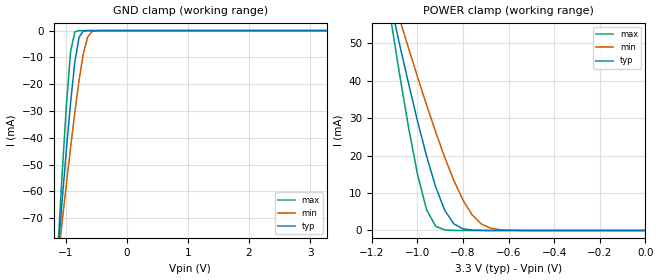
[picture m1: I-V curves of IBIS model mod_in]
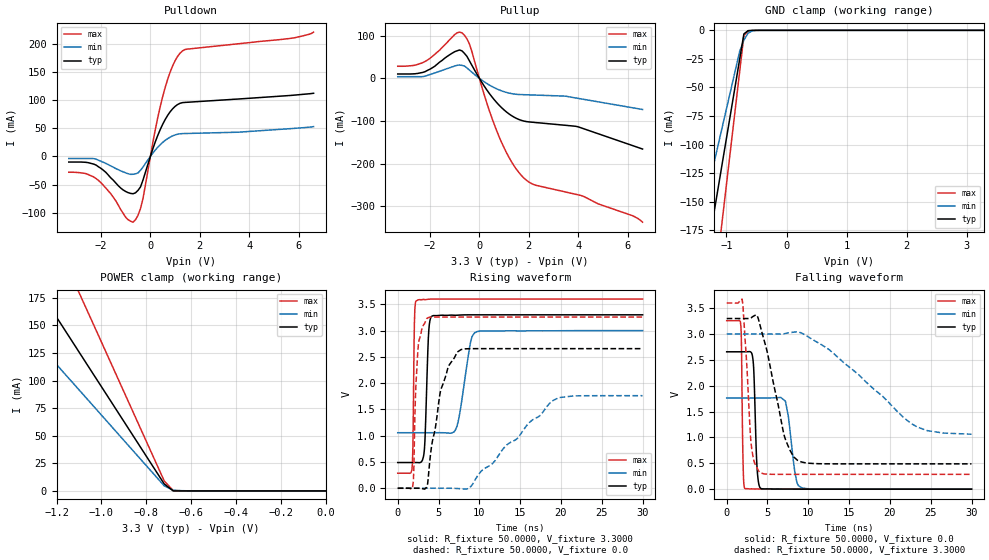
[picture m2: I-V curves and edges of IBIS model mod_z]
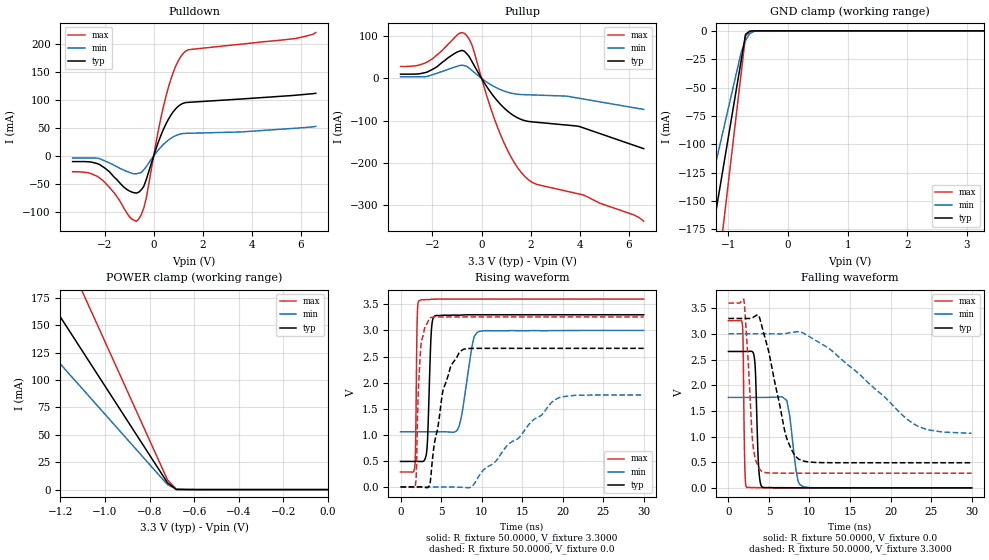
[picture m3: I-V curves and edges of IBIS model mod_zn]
| IBIS (I/O, Buffer, Information, Specification) Model, officially
| electronic behavioral standard for Buffer structures of digital pins.
[IBIS ver]  4.0
[File name] 54ac151_3v3_rev1.ibs
[File Rev]  1.0
[Date]   9 Oct 2020
[Source]   CAD & Design Services (Catania) - STMicroelectronics
[Notes]
  (Note1) This IBIS model is the model of the product with package
   (Flat16 package elements);
  (Note2) This IBIS model is extracted with nominal 3.3V power supply
   (min:3.0V, typ:3.3V, max:3.6V);
  (Note3) This model has few Warnings about the non-monotonicity
   of I-V curves, but they are not indicative of problems
   inside the model;
[Copyright] (c) 2020 STMicroelectronics
|   Component 54AC151
[Component] 54AC151
[Manufacturer] STMicroelectronics
[Package]
| variable  typ   min   max
R_pkg   0.0   0.0   0.0
L_pkg   0.0H   0.0H   0.0H
C_pkg   0.0F   0.0F   0.0F
[Pin]   signal_name   model_name   R_pin   L_pin   C_pin
1   I3   mod_in   87.8m   2.68nH   1.16pF
2   I2   mod_in   53.6m   1.94nH   1.11pF
3   I1   mod_in   34.1m   1.02nH   0.87pF
4   IO   mod_in   34.1m   1.02nH   0.87pF
5   Z   mod_z   34.1m   1.02nH   0.87pF
6   ZN   mod_zn   34.1m   1.02nH   0.87pF
7   EN   mod_en   53.6m   1.94nH   1.11pF
8   GND   GND   87.8m   2.68nH   1.16pF
9   S2   mod_s   87.8m   2.68nH   1.16pF
10   S1   mod_s   53.6m   1.94nH   1.11pF
11   S0   mod_s   34.1m   1.02nH   0.87pF
12   I7   mod_in   34.1m   1.02nH   0.87pF
13   I6   mod_in   34.1m   1.02nH   0.87pF
14   I5   mod_in   34.1m   1.02nH   0.87pF
15   I4   mod_in   53.6m   1.94nH   1.11pF
16   VCC   POWER   87.8m   2.68nH   1.16pF
| Models and submodels in the file (5): mod_in (Input), mod_z (3-state), mod_zn (3-state), mod_en (Input), mod_s (Input)
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|   Model mod_in
[Model]   mod_in
Model_type Input
Vinl   =   0.8000V
Vinh   =   2.0000V
C_comp   0.584pF   0.423pF   0.735pF
[Temperature Range]  25.0000   0.1250k   -55.0000
[Voltage Range]   3.3000V   3.0000V   3.6000V
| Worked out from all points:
|   GND clamp passes 1 mA (typ) near -0.74 V on its own axis
|   POWER clamp passes 1 mA (typ) near -0.82 V on its own axis
[GND_clamp]
|Voltage   I(typ)   I(min)   I(max)
-3.3V     -749mA     -568.4mA   -1.036A
-1.13V    -83.59mA   -86.24mA   -82mA
-1.06V    -63.75mA   -71.67mA   -54.05mA
-990mV    -44.61mA   -57.39mA   -28.12mA
-920mV    -26.72mA   -43.53mA   -7.665mA
-850mV    -11.52mA   -30.34mA   -438.9uA
-780mV    -2.357mA   -18.3mA    -11.16uA
-710mV    -202.6uA   -8.403mA   -269.9nA
-640mV    -13.61uA   -2.366mA   -6.525nA
-570mV    -893.7nA   -396.6uA   -166.8pA
-430mV    -3.851nA   -7.049uA   -9.012pA
3.28V     6.52pA     5.985nA    5.92pA
[POWER_clamp]
|Voltage   I(typ)   I(min)   I(max)
-3.28V    721.1mA    542.9mA    1.005A
-1.12V    61.08mA    64.91mA    57.6mA
-1.08V    50.1mA     56.8mA     42.24mA
-1.04V    39.44mA    48.83mA    27.8mA
-1V       29.27mA    41.04mA    15.03mA
-960mV    19.83mA    33.48mA    5.53mA
-920mV    11.6mA     26.24mA    1.117mA
-880mV    5.323mA    19.44mA    149.5uA
-840mV    1.752mA    13.28mA    18.09uA
-760mV    95.85uA    4.147mA    257.2nA
-680mV    4.309uA    632.9uA    3.657nA
0V        6.6pA      45.39pA    7.2pA
|   Model mod_z
[Model]   mod_z
Model_type 3-state
Polarity   Non-Inverting
Enable   Active-Low
| Vinl   =   0.8000V
| Vinh   =   2.0000V
Vmeas  =   1.650V
Cref   =   50pF
Rref   =   500
Vref   =   0.0
C_comp   3.207pF   2.433pF   4.228pF
[Temperature Range]  25.0000   0.1250k   -55.0000
[Voltage Range]   3.3000V   3.0000V   3.6000V
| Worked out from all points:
|   slope of the pulldown table from 0 to 0.495 V, typ, clamps not added: 8.73 ohm
|   slope of the pullup table from 0 to 0.495 V, typ, clamps not added: 11.6 ohm
|   GND clamp passes 1 mA (typ) near -0.66 V on its own axis
|   POWER clamp passes 1 mA (typ) near -0.69 V on its own axis
|   rising waveform, R_fixture 50.0000, V_fixture 3.3000: 20-80 % time 350ps typ, 1.11ns min, 147ps max; typ from 0.489 V to 3.3 V
|   rising waveform, R_fixture 50.0000, V_fixture 0.0: 20-80 % time 1.92ns typ, 7.15ns min, 456ps max; typ from 0 V to 2.66 V
|   falling waveform, R_fixture 50.0000, V_fixture 0.0: 20-80 % time 316ps typ, 778ps min, 163ps max; typ from 2.66 V to 0 V
|   falling waveform, R_fixture 50.0000, V_fixture 3.3000: 20-80 % time 2.19ns typ, 8.06ns min, 717ps max; typ from 3.3 V to 0.489 V
[Pulldown]
|Voltage   I(typ)   I(min)   I(max)
-3.3V     -10.02mA   -3.72mA    -28.12mA
-2.1V     -18.41mA   -6.713mA   -42.56mA
-1.6V     -38.11mA   -16.98mA   -66.25mA
-1V       -62.22mA   -29.14mA   -107.8mA
-700mV    -66.24mA   -31.66mA   -116.7mA
-500mV    -60.23mA   -29.28mA   -104.6mA
-300mV    -42.06mA   -19.04mA   -75.1mA
200mV     25.93mA    11.34mA    47.73mA
600mV     65.52mA    28.45mA    122.5mA
900mV     84.46mA    36.38mA    160.6mA
1.2V      94.2mA     40.13mA    183.1mA
6.6V      112mA      52.87mA    220.5mA
[Pullup]
|Voltage   I(typ)   I(min)   I(max)
-3.3V     10.02mA    3.72mA     28.12mA
-2.2V     15.31mA    4.805mA    39.21mA
-1V       62.21mA    28.63mA    102.3mA
-700mV    64.18mA    30.12mA    106.5mA
-400mV    40.78mA    19.13mA    80.3mA
300mV     -27.16mA   -12.16mA   -57.61mA
800mV     -63.16mA   -27.27mA   -137.1mA
1.3V      -87.59mA   -35.96mA   -195.8mA
1.7V      -98.8mA    -38.31mA   -227.9mA
2.2V      -103.4mA   -39.31mA   -249.4mA
4V        -114mA     -47.24mA   -273.5mA
6.6V      -166mA     -73.24mA   -337.6mA
[GND_clamp]
|Voltage   I(typ)   I(min)   I(max)
-3.3V     -818.6mA   -595.5mA   -1.169A
-1.48V    -245.6mA   -178.6mA   -350.7mA
-1.41V    -223.5mA   -162.6mA   -319.2mA
-1.27V    -179.5mA   -130.5mA   -256.3mA
-1.2V     -157.4mA   -114.5mA   -224.8mA
-1.13V    -135.4mA   -98.48mA   -193.3mA
-1.06V    -113.3mA   -82.45mA   -161.9mA
-780mV    -25.19mA   -18.41mA   -35.97mA
-710mV    -3.148mA   -8.533mA   -4.496mA
-640mV    -262.4uA   -2.478mA   -621.5uA
-430mV    -2.368uA   -13.65uA   -1.116uA
3.28V     8.201nA    6.403nA    13.62nA
[POWER_clamp]
|Voltage   I(typ)   I(min)   I(max)
-3.28V    812.3mA    590.9mA    1.16A
-1.48V    245.6mA    178.6mA    350.7mA
-1.44V    233mA      169.5mA    332.7mA
-1.28V    182.6mA    132.8mA    260.8mA
-1.24V    170mA      123.7mA    242.8mA
-1.12V    132.2mA    96.19mA    188.8mA
-1.08V    119.6mA    87.03mA    170.8mA
-720mV    6.297mA    4.581mA    8.992mA
-680mV    11.43uA    625.6uA    325uA
0V        0A         0A         0A
[Ramp]
| variable   typ   min   max
dV/dt_r   1.5939/1.9165n  1.0412/7.0920n  1.9546/0.4951n
dV/dt_f   1.6866/2.1980n  0.8156/5.9356n  1.9880/0.7318n
R_load = 50.0000
[Rising Waveform]
R_fixture= 50.0000
V_fixture= 3.3000
V_fixture_min= 3.0000
V_fixture_max= 3.6000
|time   V(typ)   V(min)   V(max)
0s        489.4mV    1.057V     286.6mV
1.74ns    489.4mV    1.057V     352.9mV
2.04ns    489.4mV    1.057V     3.119V
2.22ns    489.5mV    1.057V     3.56V
3.21ns    652.8mV    1.057V     3.593V
3.81ns    3.011V     1.057V     3.597V
4.2ns     3.276V     1.057V     3.6V
7.05ns    3.292V     1.103V     3.6V
9.72ns    3.3V       2.981V     3.6V
30ns      3.3V       3V         3.6V
[Rising Waveform]
R_fixture= 50.0000
V_fixture= 0.0
V_fixture_min= 0.0
V_fixture_max= 0.0
|time   V(typ)   V(min)   V(max)
0s        0V         0V         0V
1.83ns    -688.9nV   -2.461uV   29.32mV
1.98ns    -2.667uV   -1.585uV   405.2mV
2.22ns    61.06uV    -397.4nV   1.934V
2.52ns    369.1uV    19.53nV    2.718V
3.66ns    83.21mV    -186.4nV   3.241V
5.28ns    1.878V     17.22uV    3.258V
7.77ns    2.639V     -9.254mV   3.258V
18.93ns   2.657V     1.662V     3.258V
30ns      2.657V     1.762V     3.258V
[Falling Waveform]
R_fixture= 50.0000
V_fixture= 0.0
V_fixture_min= 0.0
V_fixture_max= 0.0
|time   V(typ)   V(min)   V(max)
0s        2.657V     1.762V     3.258V
1.74ns    2.656V     1.762V     3.151V
2.01ns    2.657V     1.762V     494.3mV
2.25ns    2.657V     1.762V     10.64mV
3.21ns    2.521V     1.761V     5.356mV
3.72ns    417.3mV    1.761V     4.585mV
4.17ns    16.08mV    1.762V     2.218mV
7.2ns     2.198mV    1.701V     1.387uV
9.24ns    811uV      21.88mV    -39.46nV
30ns      -447.8pV   31.63uV    -48.54nV
[Falling Waveform]
R_fixture= 50.0000
V_fixture= 3.3000
V_fixture_min= 3.0000
V_fixture_max= 3.6000
|time   V(typ)   V(min)   V(max)
0s        3.3V       3V         3.6V
1.89ns    3.3V       3V         3.676V
2.4ns     3.3V       3V         2.566V
3ns       3.313V     3V         874.7mV
3.36ns    3.352V     3V         534.6mV
4.11ns    3.158V     3V         322.5mV
7.05ns    1.038V     3.006V     286.7mV
8.67ns    559.3mV    3.044V     286.6mV
22.74ns   489.4mV    1.257V     286.6mV
30ns      489.4mV    1.063V     286.6mV
|   Model mod_zn
[Model]   mod_zn
Model_type 3-state
Polarity   Inverting
Enable   Active-Low
| Vinl   =   0.8000V
| Vinh   =   2.0000V
Vmeas  =   1.650V
Cref   =   50pF
Rref   =   500
Vref   =   0.0
C_comp   3.207pF   2.433pF   4.228pF
[Temperature Range]  25.0000   0.1250k   -55.0000
[Voltage Range]   3.3000V   3.0000V   3.6000V
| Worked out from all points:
|   slope of the pulldown table from 0 to 0.495 V, typ, clamps not added: 8.73 ohm
|   slope of the pullup table from 0 to 0.495 V, typ, clamps not added: 11.6 ohm
|   GND clamp passes 1 mA (typ) near -0.66 V on its own axis
|   POWER clamp passes 1 mA (typ) near -0.69 V on its own axis
|   rising waveform, R_fixture 50.0000, V_fixture 3.3000: 20-80 % time 350ps typ, 1.11ns min, 147ps max; typ from 0.489 V to 3.3 V
|   rising waveform, R_fixture 50.0000, V_fixture 0.0: 20-80 % time 1.92ns typ, 7.15ns min, 456ps max; typ from 0 V to 2.66 V
|   falling waveform, R_fixture 50.0000, V_fixture 0.0: 20-80 % time 316ps typ, 778ps min, 163ps max; typ from 2.66 V to 0 V
|   falling waveform, R_fixture 50.0000, V_fixture 3.3000: 20-80 % time 2.19ns typ, 8.06ns min, 717ps max; typ from 3.3 V to 0.489 V
[Pulldown]
|Voltage   I(typ)   I(min)   I(max)
-3.3V     -10.02mA   -3.72mA    -28.12mA
-2.1V     -18.41mA   -6.713mA   -42.56mA
-1.6V     -38.11mA   -16.98mA   -66.25mA
-1V       -62.22mA   -29.14mA   -107.8mA
-700mV    -66.24mA   -31.66mA   -116.7mA
-500mV    -60.23mA   -29.28mA   -104.6mA
-300mV    -42.06mA   -19.04mA   -75.1mA
200mV     25.93mA    11.34mA    47.73mA
600mV     65.52mA    28.45mA    122.5mA
900mV     84.46mA    36.38mA    160.6mA
1.2V      94.2mA     40.13mA    183.1mA
6.6V      112mA      52.87mA    220.5mA
[Pullup]
|Voltage   I(typ)   I(min)   I(max)
-3.3V     10.02mA    3.72mA     28.12mA
-2.2V     15.31mA    4.805mA    39.21mA
-1V       62.21mA    28.63mA    102.3mA
-700mV    64.18mA    30.12mA    106.5mA
-400mV    40.78mA    19.13mA    80.3mA
300mV     -27.16mA   -12.16mA   -57.61mA
800mV     -63.16mA   -27.27mA   -137.1mA
1.3V      -87.59mA   -35.96mA   -195.8mA
1.7V      -98.8mA    -38.31mA   -227.9mA
2.2V      -103.4mA   -39.31mA   -249.4mA
4V        -114mA     -47.24mA   -273.5mA
6.6V      -166mA     -73.24mA   -337.6mA
[GND_clamp]
|Voltage   I(typ)   I(min)   I(max)
-3.3V     -818.6mA   -595.5mA   -1.169A
-1.48V    -245.6mA   -178.6mA   -350.7mA
-1.41V    -223.5mA   -162.6mA   -319.2mA
-1.27V    -179.5mA   -130.5mA   -256.3mA
-1.2V     -157.4mA   -114.5mA   -224.8mA
-1.13V    -135.4mA   -98.48mA   -193.3mA
-1.06V    -113.3mA   -82.45mA   -161.9mA
-780mV    -25.19mA   -18.41mA   -35.97mA
-710mV    -3.148mA   -8.533mA   -4.496mA
-640mV    -262.4uA   -2.478mA   -621.5uA
-430mV    -2.368uA   -13.65uA   -1.116uA
3.28V     8.201nA    6.403nA    13.62nA
[POWER_clamp]
|Voltage   I(typ)   I(min)   I(max)
-3.28V    812.3mA    590.9mA    1.16A
-1.48V    245.6mA    178.6mA    350.7mA
-1.44V    233mA      169.5mA    332.7mA
-1.28V    182.6mA    132.8mA    260.8mA
-1.24V    170mA      123.7mA    242.8mA
-1.12V    132.2mA    96.19mA    188.8mA
-1.08V    119.6mA    87.03mA    170.8mA
-720mV    6.297mA    4.581mA    8.992mA
-680mV    11.43uA    625.6uA    325uA
0V        0A         0A         0A
[Ramp]
| variable   typ   min   max
dV/dt_r   1.5939/1.9165n  1.0412/7.0920n  1.9546/0.4951n
dV/dt_f   1.6866/2.1980n  0.8156/5.9356n  1.9880/0.7318n
R_load = 50.0000
[Rising Waveform]
R_fixture= 50.0000
V_fixture= 3.3000
V_fixture_min= 3.0000
V_fixture_max= 3.6000
|time   V(typ)   V(min)   V(max)
0s        489.4mV    1.057V     286.6mV
1.74ns    489.4mV    1.057V     352.9mV
2.04ns    489.4mV    1.057V     3.119V
2.22ns    489.5mV    1.057V     3.56V
3.21ns    652.8mV    1.057V     3.593V
3.81ns    3.011V     1.057V     3.597V
4.2ns     3.276V     1.057V     3.6V
7.05ns    3.292V     1.103V     3.6V
9.72ns    3.3V       2.981V     3.6V
30ns      3.3V       3V         3.6V
[Rising Waveform]
R_fixture= 50.0000
V_fixture= 0.0
V_fixture_min= 0.0
V_fixture_max= 0.0
|time   V(typ)   V(min)   V(max)
0s        0V         0V         0V
1.83ns    -688.9nV   -2.461uV   29.32mV
1.98ns    -2.667uV   -1.585uV   405.2mV
2.22ns    61.06uV    -397.4nV   1.934V
2.52ns    369.1uV    19.53nV    2.718V
3.66ns    83.21mV    -186.4nV   3.241V
5.28ns    1.878V     17.22uV    3.258V
7.77ns    2.639V     -9.254mV   3.258V
18.93ns   2.657V     1.662V     3.258V
30ns      2.657V     1.762V     3.258V
[Falling Waveform]
R_fixture= 50.0000
V_fixture= 0.0
V_fixture_min= 0.0
V_fixture_max= 0.0
|time   V(typ)   V(min)   V(max)
0s        2.657V     1.762V     3.258V
1.74ns    2.656V     1.762V     3.151V
2.01ns    2.657V     1.762V     494.3mV
2.25ns    2.657V     1.762V     10.64mV
3.21ns    2.521V     1.761V     5.356mV
3.72ns    417.3mV    1.761V     4.585mV
4.17ns    16.08mV    1.762V     2.218mV
7.2ns     2.198mV    1.701V     1.387uV
9.24ns    811uV      21.88mV    -39.46nV
30ns      -447.8pV   31.63uV    -48.54nV
[Falling Waveform]
R_fixture= 50.0000
V_fixture= 3.3000
V_fixture_min= 3.0000
V_fixture_max= 3.6000
|time   V(typ)   V(min)   V(max)
0s        3.3V       3V         3.6V
1.89ns    3.3V       3V         3.676V
2.4ns     3.3V       3V         2.566V
3ns       3.313V     3V         874.7mV
3.36ns    3.352V     3V         534.6mV
4.11ns    3.158V     3V         322.5mV
7.05ns    1.038V     3.006V     286.7mV
8.67ns    559.3mV    3.044V     286.6mV
22.74ns   489.4mV    1.257V     286.6mV
30ns      489.4mV    1.063V     286.6mV
